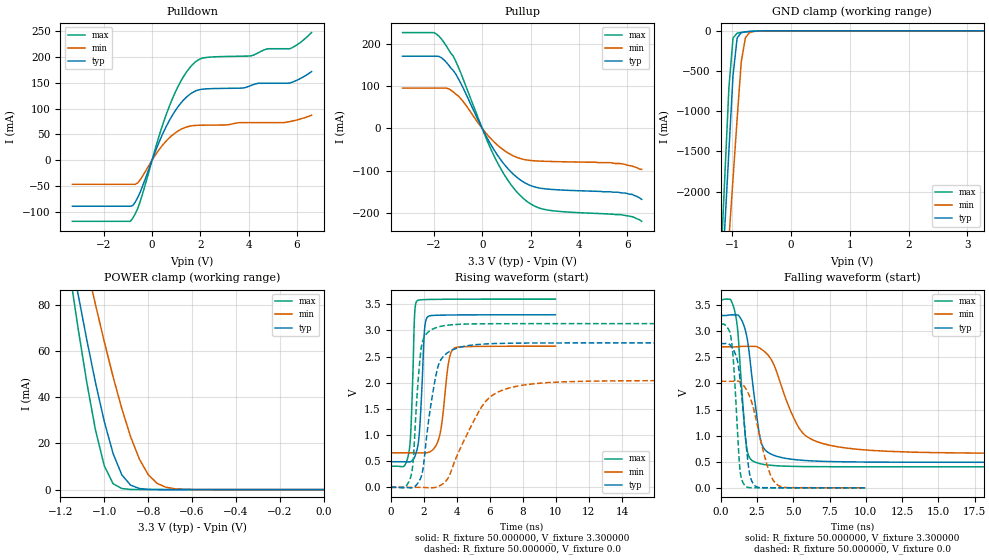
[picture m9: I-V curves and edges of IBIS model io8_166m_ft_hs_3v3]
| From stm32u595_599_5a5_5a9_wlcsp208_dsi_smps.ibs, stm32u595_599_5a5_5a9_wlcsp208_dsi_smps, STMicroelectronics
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|   Model io8_166m_ft_hs_3v3
[Model]  io8_166m_ft_hs_3v3
Model_type I/O
Polarity   Non-Inverting
Enable   Active-Low
Vinl =   0.990000V
Vinh =   2.310000V
Vmeas =  1.650000V
Cref =   50.000000pF
Rref =   100.000000M
Vref =   0.0V
C_comp   3.517200pF   3.489400pF   3.557800pF
[Temperature Range]   25.000000   0.140000k   -40.000000
[Pullup Reference]   3.300000V   2.700000V   3.600000V
[Pulldown Reference]   0.0V   0.0V   0.0V
[POWER Clamp Reference]   3.300000V   2.700000V   3.600000V
[GND Clamp Reference]   0.0V   0.0V   0.0V
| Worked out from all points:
|   slope of the pulldown table from 0 to 0.495 V, typ, clamps not added: 8.73 ohm
|   slope of the pullup table from 0 to 0.495 V, typ, clamps not added: 9.64 ohm
|   GND clamp passes 1 mA (typ) near -0.50 V on its own axis
|   POWER clamp passes 1 mA (typ) near -0.85 V on its own axis
|   rising waveform, R_fixture 50.000000, V_fixture 3.300000: 20-80 % time 260ps typ, 443ps min, 195ps max; typ from 0.49 V to 3.3 V
|   rising waveform, R_fixture 50.000000, V_fixture 0.0: 20-80 % time 750ps typ, 1.95ns min, 402ps max; typ from 0 V to 2.76 V
|   falling waveform, R_fixture 50.000000, V_fixture 3.300000: 20-80 % time 759ps typ, 1.84ns min, 492ps max; typ from 3.3 V to 0.49 V
|   falling waveform, R_fixture 50.000000, V_fixture 0.0: 20-80 % time 576ps typ, 1.09ns min, 397ps max; typ from 2.76 V to 0 V
[Pulldown]
|Voltage   I(typ)   I(min)   I(max)
-3.3V     -89.72mA   -47.06mA   -119mA
-900mV    -89.72mA   -47.06mA   -119mA
-500mV    -62.92mA   -38.71mA   -81.44mA
300mV     36.2mA     21.01mA    48.7mA
800mV     84.07mA    46.96mA    114.8mA
1.3V      116.7mA    62.09mA    162.4mA
1.8V      134.4mA    67.39mA    191.2mA
2.3V      138.6mA    67.98mA    199.8mA
4.1V      145.2mA    72.79mA    202.7mA
4.8V      149.4mA    72.79mA    216.5mA
5.7V      149.8mA    74.8mA     216.5mA
6.6V      172mA      87.1mA     247.9mA
[Pullup]
|Voltage   I(typ)   I(min)   I(max)
-3.3V     171.2mA    95.79mA    227.3mA
-2V       171.2mA    95.79mA    227.1mA
-1.6V     163.4mA    95.79mA    205.2mA
-1V       119.2mA    77.42mA    146.9mA
100mV     -11.39mA   -7.258mA   -14.51mA
600mV     -60.65mA   -37.83mA   -77.69mA
1.2V      -103.6mA   -62.35mA   -134mA
1.8V      -129.9mA   -74.33mA   -170.6mA
2.7V      -143.6mA   -78mA      -193.3mA
5.6V      -151mA     -83mA      -204mA
6.2V      -156mA     -89mA      -209mA
6.6V      -168mA     -97mA      -220mA
[GND_clamp]
|Voltage   I(typ)   I(min)   I(max)
-3.3V     -9.098A    -9.372A    -9.671A
-1.2V     -3.386A    -4.091A    -2.933A
-1.13V    -2.437A    -3.34A     -1.815A
-1.06V    -1.49A     -2.588A    -705.6mA
-990mV    -555.7mA   -1.839A    -89.03mA
-920mV    -88.12mA   -1.093A    -28.78mA
-850mV    -22.35mA   -387.4mA   -19.84mA
-780mV    -12.12mA   -88.01mA   -13.88mA
-710mV    -7.71mA    -22.52mA   -8.846mA
-640mV    -4.545mA   -7.864mA   -4.87mA
-360mV    -31.12uA   -173.5uA   -8.497uA
3.28V     0A         14.15nA    -7.901nA
[POWER_clamp]
|Voltage   I(typ)   I(min)   I(max)
-3.28V    1.355A     1.167A     1.664A
-1.16V    105.7mA    131.6mA    95.69mA
-1.12V    84.97mA    114mA      70.27mA
-1.08V    65.05mA    96.83mA    46.54mA
-1.04V    46.34mA    80.15mA    25.76mA
-1V       29.51mA    64.13mA    10.3mA
-960mV    15.69mA    48.99mA    2.571mA
-920mV    6.373mA    35.1mA     455.6uA
-840mV    490.7uA    13.24mA    11.36uA
-760mV    27.33uA    2.767mA    278.3nA
-640mV    347.6nA    134.1uA    16.77nA
0V        0A         19.95nA    0A
[Ramp]
| variable   typ   min   max
dV/dt_r  1.65714/0.74876n   1.22454/1.94807n   1.87854/0.40111n
dV/dt_f  1.68607/0.75781n   1.22354/1.83529n   1.91789/0.49020n
R_load = 50.000000
[Rising Waveform]
R_fixture= 50.000000
V_fixture= 3.300000
V_fixture_min= 2.700000
V_fixture_max= 3.600000
|time   V(typ)   V(min)   V(max)
0s        489.9mV    659.7mV    403.5mV
1.121ns   485.6mV    659.8mV    691.5mV
1.261ns   497.6mV    659.7mV    1.343V
1.461ns   581.9mV    659.7mV    3.343V
1.602ns   721mV      659.6mV    3.566V
2.062ns   3.036V     657.9mV    3.591V
2.242ns   3.262V     664.9mV    3.592V
2.983ns   3.293V     1.008V     3.596V
3.844ns   3.296V     2.66V      3.598V
9.97ns    3.3V       2.7V       3.599V
[Rising Waveform]
R_fixture= 50.000000
V_fixture= 0.0
V_fixture_min= 0.0
V_fixture_max= 0.0
|time   V(typ)   V(min)   V(max)
0s        3.584uV    4.869uV    1.478uV
1.251ns   -9.84mV    38.93uV    236.3mV
1.351ns   -4.937mV   55.11uV    437.7mV
1.602ns   59.61mV    134.5uV    1.76V
1.852ns   202.2mV    -413.2uV   2.663V
2.753ns   2.152V     2.385mV    3.053V
3.504ns   2.587V     190.8mV    3.102V
5.606ns   2.739V     1.583V     3.128V
7.207ns   2.756V     1.902V     3.13V
24.92ns   2.762V     2.041V     3.131V
[Falling Waveform]
R_fixture= 50.000000
V_fixture= 3.300000
V_fixture_min= 2.700000
V_fixture_max= 3.600000
|time   V(typ)   V(min)   V(max)
0s        3.3V       2.7V       3.599V
1.001ns   3.312V     2.699V     3.342V
1.201ns   3.307V     2.702V     2.925V
1.752ns   2.959V     2.71V      844.2mV
2.302ns   1.775V     2.709V     501.4mV
2.703ns   972.1mV    2.673V     463.6mV
3.103ns   714.3mV    2.587V     442.7mV
5.355ns   534.3mV    1.164V     409.3mV
6.957ns   508.5mV    854.3mV    405.5mV
24.92ns   489.9mV    659.7mV    403.5mV
[Falling Waveform]
R_fixture= 50.000000
V_fixture= 0.0
V_fixture_min= 0.0
V_fixture_max= 0.0
|time   V(typ)   V(min)   V(max)
0s        2.762V     2.041V     3.131V
720.7ps   2.711V     2.041V     2.854V
920.9ps   2.621V     2.042V     2.245V
1.321ns   2.104V     2.03V      364.8mV
1.662ns   1.103V     1.928V     46.41mV
1.942ns   350.7mV    1.785V     5.296mV
2.202ns   97.29mV    1.582V     3.321mV
3.203ns   2.842mV    432.9mV    1.49mV
3.904ns   1.735mV    57.72mV    1.033mV
9.97ns    3.584uV    4.869uV    1.478uV
